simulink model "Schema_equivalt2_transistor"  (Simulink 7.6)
settings: Solver=ode15s  StartTime=0.0  StopTime=5e-3  RelTol=1e-3
InitFcn:
  | % paramètres hybrides du transistor
  | h11=1e3;
  | h12=5e-4;
  | h21=100;
  | h22=5e-5;
  | 
  | % résistances de polarisation
  | Rc=10e3;
  | Rb=47e3;
StopFcn:
  | close all
  | load es.mat
  | plotyy(x(1,:),x(2,:),x(1,:),x(3,:))
  | title('Schéma équivalent du transistor')
  | grid
libraries: fl_lib x19, nesl_utility x3

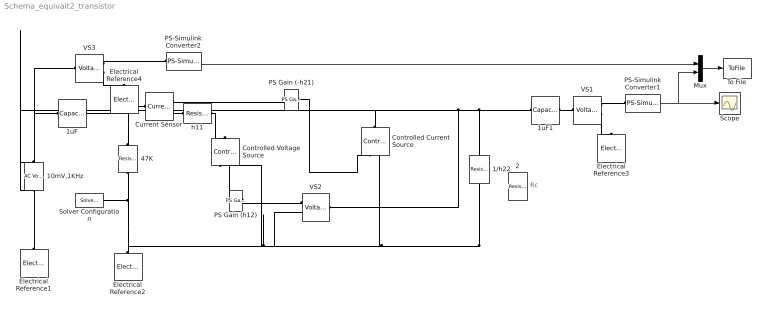
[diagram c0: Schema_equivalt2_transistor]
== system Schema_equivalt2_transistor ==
  note: Rc
  1/h22 : fl_lib/Electrical/Electrical Elements/Resistor  DialogController=NetworkEngine.DynNeDlgSource  SystemSampleTime=-1  R=1/h22 Ohm  i_Log=off  v_Log=off  LocalVarNames=|current|voltage|power  LocalVarDescs=|Resistor current (A)|Voltage across resistor (V)|Power (W)  LocalVarLogging=[0 0 0]
  10mV,1KHz : fl_lib/Electrical/Electrical Sources/AC Voltage Source  DialogController=NetworkEngine.DynNeDlgSource  SystemSampleTime=-1  amp=0.01 V  shift=0 rad  omega=1000 Hz  i_Log=off  v_Log=off  LocalVarNames=|current|voltage|power  LocalVarDescs=|Current (A)|Voltage (V)|Power (W)  LocalVarLogging=[0 0 0]
  1uF : fl_lib/Electrical/Electrical Elements/Capacitor  DialogController=NetworkEngine.DynNeDlgSource  SystemSampleTime=-1  c=1e-06 F  v0=0 V  r=1e-06 Ohm  g=0 1/Ohm  i_Log=off  v_Log=off  vc_Log=off  LocalVarNames=|current|voltage|power  LocalVarDescs=|Capacitor current (A)|Voltage across capacitor (V)|Power (W)  LocalVarLogging=[0 0 0]
  1uF1 : fl_lib/Electrical/Electrical Elements/Capacitor  DialogController=NetworkEngine.DynNeDlgSource  SystemSampleTime=-1  c=1e-06 F  v0=0 V  r=1e-06 Ohm  g=0 1/Ohm  i_Log=off  v_Log=off  vc_Log=off  LocalVarNames=|current|voltage|power  LocalVarDescs=|Capacitor current (A)|Voltage across capacitor (V)|Power (W)  LocalVarLogging=[0 0 0]
  2 : fl_lib/Electrical/Electrical Elements/Resistor  DialogController=NetworkEngine.DynNeDlgSource  SystemSampleTime=-1  R=Rc Ohm  i_Log=off  v_Log=off  LocalVarNames=|current|voltage|power  LocalVarDescs=|Resistor current (A)|Voltage across resistor (V)|Power (W)  LocalVarLogging=[0 0 0]
  47K : fl_lib/Electrical/Electrical Elements/Resistor  DialogController=NetworkEngine.DynNeDlgSource  SystemSampleTime=-1  R=Rb Ohm  i_Log=off  v_Log=off  LocalVarNames=|current|voltage|power  LocalVarDescs=|Resistor current (A)|Voltage across resistor (V)|Power (W)  LocalVarLogging=[0 0 0]
  Controlled Current Source : fl_lib/Electrical/Electrical Sources/Controlled Current Source  DialogController=NetworkEngine.DynNeDlgSource  SystemSampleTime=-1  i_Log=off  v_Log=off  LocalVarNames=|i|v  LocalVarDescs=|i|v  LocalVarLogging=[0 0]
  Controlled Voltage Source : fl_lib/Electrical/Electrical Sources/Controlled Voltage Source  DialogController=NetworkEngine.DynNeDlgSource  SystemSampleTime=-1  i_Log=off  v_Log=off  LocalVarNames=|i|v  LocalVarDescs=|i|v  LocalVarLogging=[0 0]
  Current Sensor : fl_lib/Electrical/Electrical Sensors/Current Sensor  DialogController=NetworkEngine.DynNeDlgSource  SystemSampleTime=-1  i1_Log=off  v1_Log=off  LocalVarNames=|i1|v1  LocalVarDescs=|i1|v1  LocalVarLogging=[0 0]
  Electrical Reference{1..4} (4 alike) : fl_lib/Electrical/Electrical Elements/Electrical Reference  DialogController=NetworkEngine.DynNeDlgSource  SystemSampleTime=-1  i_Log=off  LocalVarNames=|i  LocalVarDescs=|i  LocalVarLogging=[]
  Mux : Mux  Inputs=2
  PS Gain (-h21) : fl_lib/Physical Signals/Functions/PS Gain  DialogController=NetworkEngine.DynNeDlgSource  SystemSampleTime=-1  gain=-h21  LocalVarLogging=[]
  PS Gain (h12) : fl_lib/Physical Signals/Functions/PS Gain  DialogController=NetworkEngine.DynNeDlgSource  SystemSampleTime=-1  gain=h12  LocalVarLogging=[]
  PS-Simulink Converter1 : nesl_utility/PS-Simulink Converter  DialogController=NetworkEngine.DynNeUtilDlgSource  SystemSampleTime=-1  PhysicalDomain=network_engine_domain  LeftPortType=input  RightPortType=output  SubClassName=ps_output  Unit=1  AffineConversion=off
  PS-Simulink Converter2 : nesl_utility/PS-Simulink Converter  DialogController=NetworkEngine.DynNeUtilDlgSource  SystemSampleTime=-1  PhysicalDomain=network_engine_domain  LeftPortType=input  RightPortType=output  SubClassName=ps_output  Unit=1  AffineConversion=off
  Scope : Scope
  Solver Configuration : nesl_utility/Solver Configuration  DialogController=NetworkEngine.DynNeUtilDlgSource  SystemSampleTime=-1  PhysicalDomain=network_engine_domain  LeftPortType=input  RightPortType=generic  SubClassName=solver  Accelerate=off  Profile=off  ResidualTolerance=1e-9  MaxNonlinIter=12  MaxModeIter=2  DoFixedCost=off  UseLocalSampling=off  DoDC=off  LinearAlgebra=Sparse  LocalSolverSampleTime=.001  LocalSolverChoice=NE_BACKWARD_EULER_ADVANCER  UseLocalSolver=off
  To File : ToFile  Filename=es  MatrixName=x
  VS1 : fl_lib/Electrical/Electrical Sensors/Voltage Sensor  DialogController=NetworkEngine.DynNeDlgSource  SystemSampleTime=-1  i1_Log=off  v1_Log=off  LocalVarNames=|i1|v1  LocalVarDescs=|i1|v1  LocalVarLogging=[]
  VS2 : fl_lib/Electrical/Electrical Sensors/Voltage Sensor  DialogController=NetworkEngine.DynNeDlgSource  SystemSampleTime=-1  i1_Log=off  v1_Log=off  LocalVarNames=|i1|v1  LocalVarDescs=|i1|v1  LocalVarLogging=[]
  VS3 : fl_lib/Electrical/Electrical Sensors/Voltage Sensor  DialogController=NetworkEngine.DynNeDlgSource  SystemSampleTime=-1  i1_Log=off  v1_Log=off  LocalVarNames=|i1|v1  LocalVarDescs=|i1|v1  LocalVarLogging=[]
  h11 : fl_lib/Electrical/Electrical Elements/Resistor  DialogController=NetworkEngine.DynNeDlgSource  SystemSampleTime=-1  R=h11 Ohm  i_Log=off  v_Log=off  LocalVarNames=|current|voltage|power  LocalVarDescs=|Resistor current (A)|Voltage across resistor (V)|Power (W)  LocalVarLogging=[0 0 0]
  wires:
  PS-Simulink Converter1/1 -> Scope/1, Mux/2
  PS-Simulink Converter2/1 -> Mux/1
  Mux/1 -> To File/1
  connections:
  10mV,1KHz/RConn1 -- Electrical Reference1/LConn1
  10mV,1KHz/LConn1 -- 1uF/LConn1 -- VS3/LConn1
  1/h22/RConn1 -- 2/LConn1 -- Solver Configuration/RConn1 -- 47K/RConn1 -- Electrical Reference2/LConn1 -- Controlled Voltage Source/RConn2 -- VS2/RConn2 -- Controlled Current Source/RConn2
  h11/RConn1 -- Controlled Voltage Source/LConn1
  1/h22/LConn1 -- 2/RConn1 -- 1uF1/LConn1 -- VS2/LConn1 -- Controlled Current Source/LConn1
  PS Gain (h12)/RConn1 -- Controlled Voltage Source/RConn1
  PS Gain (h12)/LConn1 -- VS2/RConn1
  47K/LConn1 -- 1uF/RConn1 -- Current Sensor/LConn1
  Current Sensor/RConn2 -- h11/LConn1
  PS Gain (-h21)/LConn1 -- Current Sensor/RConn1
  PS Gain (-h21)/RConn1 -- Controlled Current Source/RConn1
  VS1/RConn1 -- PS-Simulink Converter1/LConn1
  VS1/RConn2 -- Electrical Reference3/LConn1
  1uF1/RConn1 -- VS1/LConn1
  VS3/RConn2 -- Electrical Reference4/LConn1
  VS3/RConn1 -- PS-Simulink Converter2/LConn1
